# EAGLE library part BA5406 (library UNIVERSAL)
12V/5W DUAL POWER AMPLIFIER BA5406 Manufacturer ROHM.
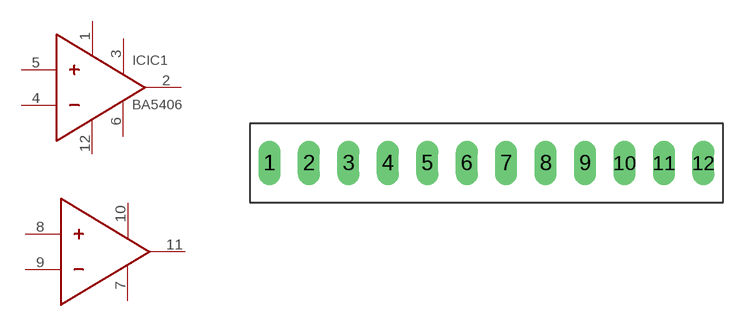
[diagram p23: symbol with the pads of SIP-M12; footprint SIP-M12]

Designator prefix IC; gates IC1=BA5406 G$2=BA5406X

## BA5406  [SIP-M12]
1  IC1:1
2  IC1:2
3  IC1:3
4  IC1:4
5  IC1:5
6  IC1:6
7  G$2:7
8  G$2:8
9  G$2:9
10  G$2:10
11  G$2:11
12  IC1:12

## Footprint SIP-M12 (pad centres in mm)
drill 0.8 pad 1.422 long: 1 0,0; 2 2.54,0; 3 5.08,0; 4 7.62,0; 5 10.16,0; 6 12.7,0; 7 15.24,0; 8 17.78,0; 9 20.32,0; 10 22.86,0; 11 25.4,0; 12 27.94,0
